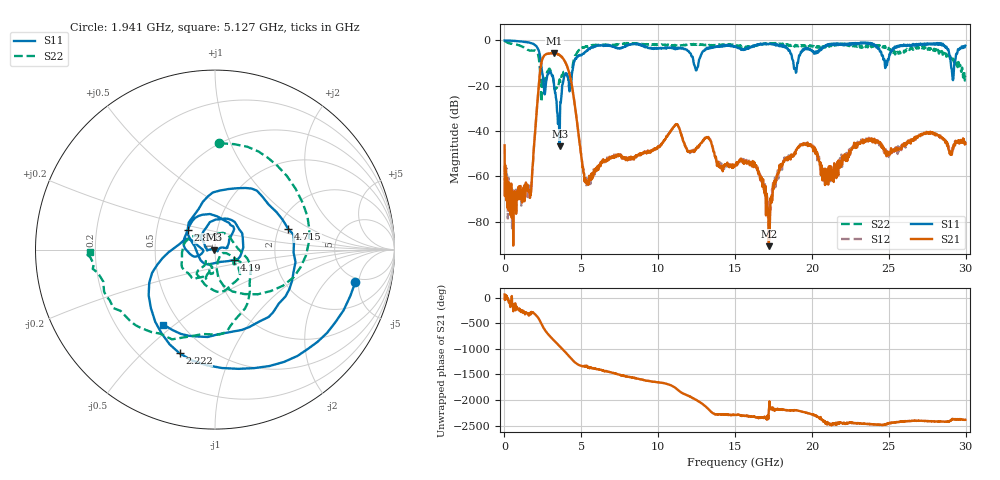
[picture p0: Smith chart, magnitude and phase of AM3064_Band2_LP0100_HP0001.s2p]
# Hz S DB R 50.0
!freq dBS11 angS11 dBS21 angS21 dBS12 angS12 dBS22 angS22
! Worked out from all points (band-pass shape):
!   1600 points, 10 MHz to 29.98 GHz, reference 50 ohm
!   highest |S21| = -5.54 dB at 3.234 GHz (marker M1); lowest = -90.7 dB at 17.2 GHz (marker M2)
!   |S21| within 3 dB of the highest: 2.449 GHz to 3.868 GHz (1.419 GHz wide, 44.9 % of centre)
!   lowest |S11| = -46.8 dB at 3.59 GHz (marker M3), VSWR 1.01, Z = 49.6 - j0.11 ohm
!   |S11| at or under -10 dB: 2.38 GHz to 4.506 GHz (2.127 GHz wide, 61.8 % of centre); 12.31 GHz to 12.62 GHz (307.2 MHz wide, 2.46 % of centre); 18.8 GHz to 19.05 GHz (250.5 MHz wide, 1.32 % of centre)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
!   |S22| runs from -27.1 to -0.2 dB; largest |S21 - S12| = 0.012
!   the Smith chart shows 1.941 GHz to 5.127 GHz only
!   S11 on the Smith chart (normalised r, x): 1.941 GHz: 4.44, -4.51; 2.222 GHz: 0.35, -0.65; 2.878 GHz: 0.72, +0.16; 4.19 GHz: 1.22, -0.15; 4.715 GHz: 2.25, +0.63; 5.127 GHz: 0.40, -0.46
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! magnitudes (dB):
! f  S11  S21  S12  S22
! 10 MHz  0.0  -46.3  -55.2  -0.2
! 609.8 MHz  -0.2  -68.0  -66.1  -1.7
! 1.641 GHz  -1.0  -66.6  -67.7  -4.5
! 1.941 GHz  -1.9  -45.1  -45.2  -4.5
! 2.222 GHz  -4.3  -20.9  -20.8  -7.4
! 2.878 GHz  -14.5  -5.8  -5.7  -12.8
! 3.234 GHz  -20.3  -5.5  -5.6  -20.7
! 3.59 GHz  -46.8  -6.5  -6.6  -17.2
! 4.19 GHz  -18.4  -13.7  -13.8  -20.0
! 4.715 GHz  -7.5  -35.7  -35.5  -5.4
! 5.015 GHz  -6.5  -52.2  -51.7  -3.8
! 5.127 GHz  -5.9  -57.8  -56.5  -3.2
! 10 GHz  -3.5  -46.6  -46.9  -1.8
! 11.2 GHz  -3.6  -37.1  -37.0  -2.3
! 15 GHz  -2.6  -55.5  -55.1  -2.0
! 16.32 GHz  -2.3  -55.5  -55.0  -2.1
! 17.2 GHz  -1.5  -90.7  -73.4  -1.7
! 18.23 GHz  -3.1  -52.8  -53.3  -1.6
! 19.99 GHz  -4.3  -47.0  -46.8  -2.3
! 20.89 GHz  -2.1  -63.5  -59.6  -2.9
! 25 GHz  -8.0  -49.3  -51.4  -3.3
! 29.98 GHz  -2.3  -45.6  -45.4  -15.8
